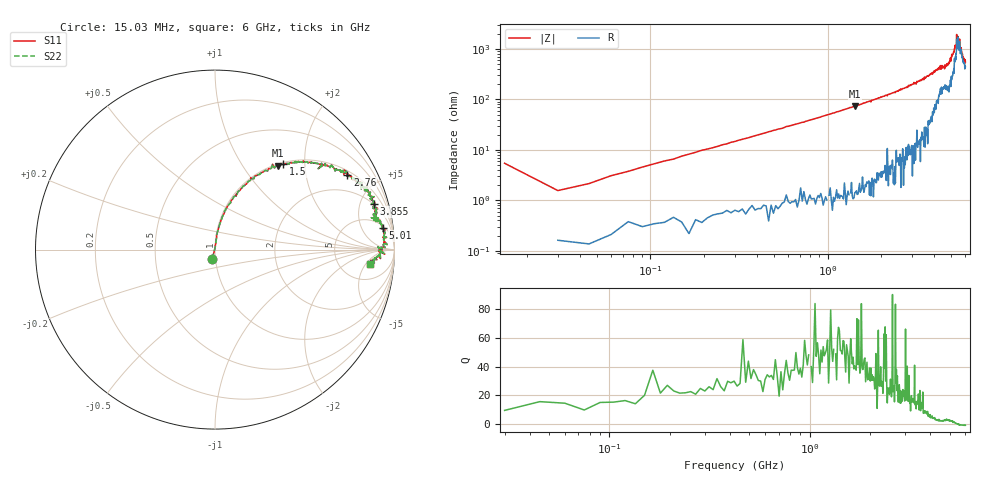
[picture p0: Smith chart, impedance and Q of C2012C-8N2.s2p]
!	Network	Analyzer	HP8753E.07.74:	Oct	30	2002	Serial	No.	JP38451487
!	Hewlett-Packard
!	7	Sep	2009	10:43:13
!	Frequency	S11	S21	S12	S22
#	HZ	S	RI	R	50
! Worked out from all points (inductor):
!   400 points, 15.03 MHz to 6 GHz, reference 50 ohm
!   read as one part in series: L = 7.94 nH near 45.03 MHz
!   highest Q = 57.6 at 1.425 GHz (marker M1), where L = 8.13 nH
!   self-resonance near 5.516 GHz
!   S11 on the Smith chart (normalised r, x): 15.03 MHz: 0.96, -0.10; 1.5 GHz: 1.03, +1.56; 2.76 GHz: 1.16, +3.43; 3.855 GHz: 1.92, +6.57; 5.01 GHz: 6, +13; 6 GHz: 10, -7
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1.502992e7  -0.0152 -0.0525  1.02 0.0525  1.02 0.0525  -0.0152 -0.0525
3.002985e7  0.00171 0.0155  0.998 -0.0155  0.998 -0.0155  0.00171 0.0155
6.00297e7  0.00308 0.0306  0.997 -0.0306  0.997 -0.0306  0.00308 0.0306
1.200294e8  0.00746 0.0596  0.993 -0.0596  0.993 -0.0596  0.00746 0.0596
2.850286e8  0.0248 0.137  0.975 -0.137  0.975 -0.137  0.0248 0.137
1.020025e9  0.21 0.395  0.79 -0.395  0.79 -0.395  0.21 0.395
1.425023e9  0.349 0.467  0.651 -0.467  0.651 -0.467  0.349 0.467
1.500022e9  0.381 0.475  0.619 -0.475  0.619 -0.475  0.381 0.475
2.01002e9  0.551 0.481  0.449 -0.481  0.449 -0.481  0.551 0.481
2.760016e9  0.737 0.417  0.263 -0.417  0.263 -0.417  0.737 0.417
3.015015e9  0.798 0.394  0.202 -0.394  0.202 -0.394  0.798 0.394
3.855011e9  0.887 0.254  0.113 -0.254  0.113 -0.254  0.887 0.254
4.00501e9  0.903 0.231  0.0974 -0.231  0.0974 -0.231  0.903 0.231
5.010005e9  0.936 0.121  0.0642 -0.121  0.0642 -0.121  0.936 0.121
5.325003e9  0.939 0.0555  0.061 -0.0555  0.061 -0.0555  0.939 0.0555
5.355003e9  0.959 0.0279  0.0407 -0.0279  0.0407 -0.0279  0.959 0.0279
5.385003e9  0.942 0.0429  0.0576 -0.0429  0.0576 -0.0429  0.942 0.0429
5.445003e9  0.948 0.0117  0.0519 -0.0117  0.0519 -0.0117  0.948 0.0117
5.535002e9  0.907 0.0152  0.0934 -0.0152  0.0934 -0.0152  0.907 0.0152
5.565002e9  0.946 -0.0254  0.0541 0.0254  0.0541 0.0254  0.946 -0.0254
5.595002e9  0.911 -0.00348  0.0891 0.00348  0.0891 0.00348  0.911 -0.00348
6e9  0.865 -0.0801  0.135 0.0801  0.135 0.0801  0.865 -0.0801
